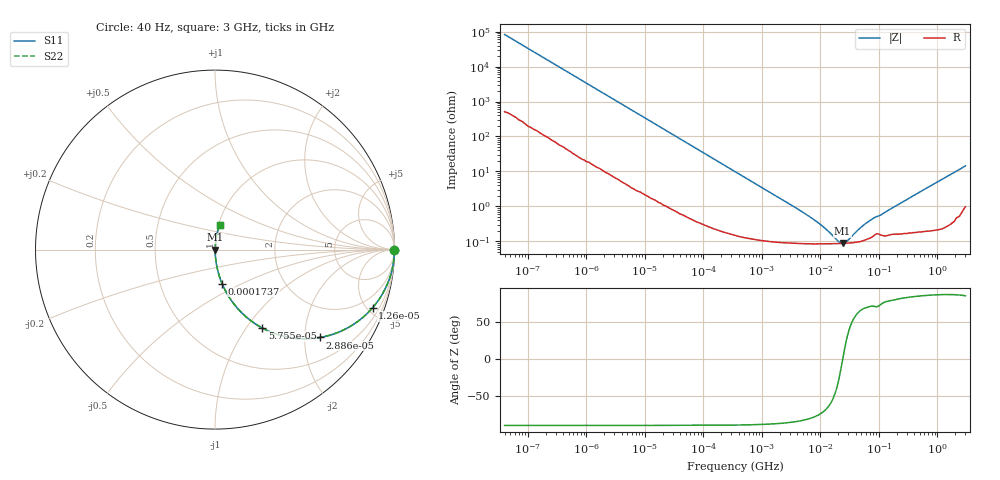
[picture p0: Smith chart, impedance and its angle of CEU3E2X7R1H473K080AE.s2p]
! S-parameter Generated by TDK Corporation
! Copyright(C) 2015 TDK Corporation.
! All Rights Reserved.
! TDK P/N: CEU3E2X7R1H473K080AE (Multilayer Ceramic Chip Capacitors)
! Property: C=47nF
! Size(LxWxT): 1.6x0.8x0.8mm, 0.063x0.031x0.031inches
! Model Type: s2p (Touchstone File Format Version 1.0)
! Frequency: DC=Yes Start=0.00004MHz Stop=3000MHz 396points Log-sweep
! Note: This model was converted from impedance.
! Model Generated on Jun. 23, 2015
! Hash(MD5):
! Port Assignments:
!  1 ---| |--- 2
! Applicable Conditions:
!  Temperature = 25 degC
!  DC Bias Voltage = 0 V
!  Small Signal Operation
! Terms and conditions regarding TDK Simulation Models
! (1)This simulation model is being provided solely for informational purposes. Please refer to the specifications of the products in terms of detailed characteristics of such products.
! (2)In no event shall TDK Corporation of any of its subsidiaries be liable for any loss or damage arising, directly or indirectly,
!  From any information contained in this simulation model, including, but not limited to loss or damages arising from any inaccuracies, omissions or errors in connection with such information.
! (3)Any and all copyrights on this simulation model are owned by TDK Corporation.
!  Duplication or redistribution of this simulation model without prior written permission from TDK Corporation is prohibited.
! (4)This simulation model is subject to any modification or change without any prior notice.
! (5)Neither TDK Corporation nor any of its subsidiaries shall make any warranty, express or implied,
!  Including but not limited to the correctness, implied warranties of merchantability and fitness for a particular purpose with respect to this simulation models.
! (6)The use of this simulation model shall be deemed to have consented to the terms and conditions hereof.
# MHz S MA R 50
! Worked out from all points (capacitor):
!   395 points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, 40 Hz to 3 GHz, reference 50 ohm
!   read as one part in series: C = 47.7 nF near 41.88 Hz
!   lowest |Z| = 86.5 mohm at 23.9 MHz (marker M1)
!   series resonance near 23.98 MHz, so ESL is about 920 pH
!   S11 on the Smith chart (normalised r, x): 40 Hz: open; 12.6 kHz: 1.03, -5.40; 28.86 kHz: 1.02, -2.37; 57.55 kHz: 1.01, -1.19; 173.7 kHz: 1.00, -0.40; 3 GHz: 1.02, +0.29
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4e-05  1 -0.1  0.001196 89.6  0.001196 89.6  1 -0.1
0.000834128  0.9996 -1.4  0.02474 88.3  0.02474 88.3  0.9996 -1.4
0.003988472  0.9925 -6.7  0.1168 83.0  0.1168 83.0  0.9925 -6.7
0.007596806  0.9747 -12.6  0.2178 77.1  0.2178 77.1  0.9747 -12.6
0.01260356  0.9359 -20.3  0.3465 69.4  0.3465 69.4  0.9359 -20.3
0.01739424  0.8884 -27.0  0.4534 62.7  0.4534 62.7  0.8884 -27.0
0.02885808  0.7613 -40.0  0.6432 49.6  0.6432 49.6  0.7613 -40.0
0.0398272  0.6492 -49.1  0.756 40.5  0.756 40.5  0.6492 -49.1
0.05755453  0.5097 -58.9  0.8565 30.6  0.8565 30.6  0.5097 -58.9
0.09548642  0.3374 -69.8  0.9385 19.7  0.9385 19.7  0.3374 -69.8
0.1736915  0.1941 -78.2  0.9789 11.2  0.9789 11.2  0.1941 -78.2
0.3464102  0.09916 -83.5  0.9936 5.7  0.9936 5.7  0.09916 -83.5
1.094655  0.03167 -86.3  0.9985 1.8  0.9985 1.8  0.03167 -86.3
7.22376  0.004481 -79.0  0.9992 0.3  0.9992 0.3  0.004481 -79.0
12.54911  0.002188 -67.4  0.9992 0.1  0.9992 0.1  0.002188 -67.4
19.88326  0.001013 -32.6  0.9991 0.0  0.9991 0.0  0.001013 -32.6
23.90217  0.0008639 -0.6  0.9991 0.0  0.9991 0.0  0.0008639 -0.6
27.44099  0.0009558 24.3  0.9991 -0.0  0.9991 -0.0  0.0009558 24.3
60.0049  0.003255 69.7  0.9989 -0.2  0.9989 -0.2  0.003255 69.7
150.6385  0.008008 78.7  0.9985 -0.5  0.9985 -0.5  0.008008 78.7
949.3681  0.04732 84.8  0.9968 -2.7  0.9968 -2.7  0.04732 84.8
3000  0.1413 78.1  0.9806 -8.1  0.9806 -8.1  0.1413 78.1
